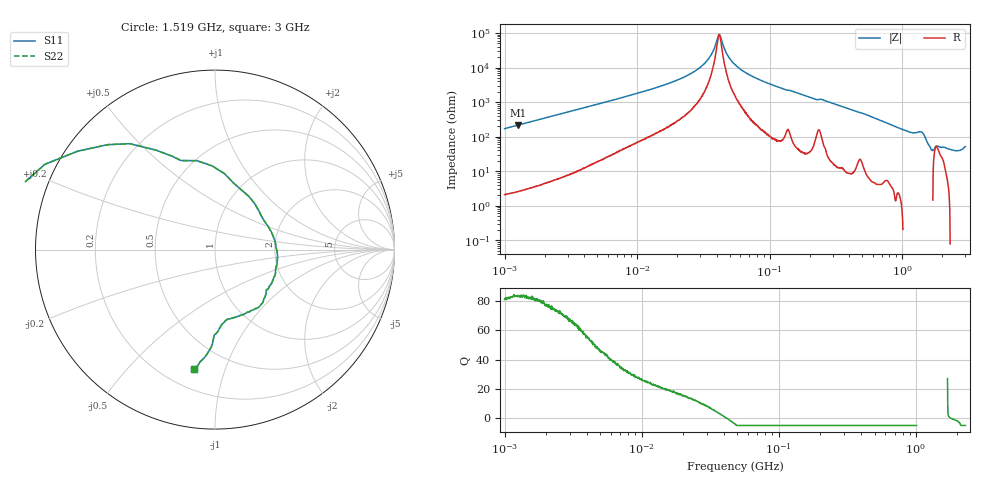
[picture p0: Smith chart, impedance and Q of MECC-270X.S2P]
!s-Parameter Generated by FASTRON Sdn. Bhd.
!FASTRON P/N : MECC-270X
!Keysight Technologies,E4991B,MY54100416,A.01.15
!Date: Thu Aug 20 11:51:47 2026
!Version  : Rev00 Thu Aug 20 11:51:47 2026
!Data & Calibration Information:
!PortZ  Port1:50+j0  Port2:50+j0
!When reading, reference impedance value at option line is always used.
!Remarks : This data is being provided solely for informational purposes.
!Freq	S11	S21	S12	S22
# Hz S dB R 50
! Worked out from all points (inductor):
!   1601 points, 1 MHz to 3 GHz, reference 50 ohm
!   read as one part in series: L = 27.2 uH near 1.041 MHz
!   highest Q = 83.7 at 1.271 MHz (marker M1), where L = 27.3 uH
!   self-resonance near 41.59 MHz
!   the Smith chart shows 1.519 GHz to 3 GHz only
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1000000  -1.32 30.1  -5.99 -59.2  -5.99 -59.2  -1.32 30.1
1271492  -0.87 24.5  -7.63 -64.8  -7.63 -64.8  -0.87 24.5
3804036  -0.12 8.7  -16.45 -80.4  -16.45 -80.4  -0.12 8.7
1.447069e7  -0.02 2.1  -28.85 -85.1  -28.85 -85.1  -0.02 2.1
3.019602e7  -0.01 0.5  -40.43 -82.3  -40.43 -82.3  -0.01 0.5
4.159437e7  -0.01 0.0  -59.21 -1.6  -59.21 -1.6  -0.01 0.0
5.477226e7  -0.01 -0.5  -41.73 82.3  -41.73 82.3  -0.01 -0.5
2.083556e8  -0.05 -4.3  -22.48 83.8  -22.48 83.8  -0.05 -4.3
7.925923e8  -0.77 -22.7  -8.27 66.2  -8.27 66.2  -0.77 -22.7
1.294266e9  -1.29 -40.1  -3.72 58.5  -3.72 58.5  -1.29 -40.1
1.374365e9  0.47 -43.0  -2.44 72.4  -2.44 72.4  0.47 -43.0
1.423359e9  2.61 -50.1  0.38 82.6  0.38 82.6  2.61 -50.1
1.466741e9  5.56 -63.8  4.66 84.5  4.66 84.5  5.56 -63.8
1.496395e9  7.96 -89.6  8.58 68.6  8.58 68.6  7.96 -89.6
1.534307e9  7.33 -138.7  9.95 29.2  9.95 29.2  7.33 -138.7
1.57318e9  3.61 -173.0  8.00 4.2  8.00 4.2  3.61 -173.0
1.604986e9  1.00 160.3  6.41 -10.4  6.41 -10.4  1.00 160.3
1.645649e9  -3.82 120.6  3.16 -22.6  3.16 -22.6  -3.82 120.6
1.704314e9  -8.76 66.5  -0.75 -21.4  -0.75 -21.4  -8.76 66.5
1.782824e9  -9.41 7.1  -3.54 -3.6  -3.54 -3.6  -9.41 7.1
1.980367e9  -8.65 -39.8  -2.45 18.3  -2.45 18.3  -8.65 -39.8
3e9  -3.40 -100.2  2.29 30.7  2.29 30.7  -3.40 -100.2
